FUNCTION_BLOCK "WEST_UHC126U_PFN"
TITLE =PN Driver
AUTHOR : 'W.E.St.'
VERSION : 1.1


VAR_INPUT
  DIRECT : BOOL ;	//Direktmodus (Sollwerte) / Direct mode for command position
  FF_ENABLE : BOOL ;	//Aktivierung der Vorsteuerung / Activation of the speed intrusion
  A_ENABLE : BOOL ;	//Aktivierung Beschleunigungsrückführung / Activation of the active damping press
  HAND_B : BOOL ;	//Handbefehl B / Manual command B
  HAND_A : BOOL ;	//Handbefehl A / Manual command A
  START : BOOL ;	//Startsignal Positionieren / Start positioning
  ENABLE : BOOL ;	//Freigabe / Unblocking
  PQ_ONLY : BOOL ;	//Deaktivierung Positionsregelung / deactivate position control
  PQ_SEL : BOOL ;	//Umschaltung zwischen Parametersatz 1 (false) und 2 (true) / Switching between p
  PQ_INVERSE : BOOL ;	//Umkehrung der Wirkrichtung des Druckreglers / Inverse mode of the pressure limi
  PQ_ACTIVE : BOOL ;	//Aktivieren des Druckreglers / Activation of the pressure limitation control
  DC_F_POS : BOOL ;	//Feinpositionierung / Fine positioning
  DC_ACTIVE : BOOL ;	//Driftkompensation / Drift compensation
  DC_FREEZE : BOOL ;	//Driftkompensation halten / Hold drift compensation value
  WA1 : REAL ;	//Sollposition 1 [mm] / Command position 1
  VA1 : REAL  := 1.000000e+002;	//Sollgeschwindigkeit 1 [%] / Command speed 1
  WA2 : REAL ;	//Sollposition 2 [mm] / Command position 2
  VA2 : REAL ;	//Sollgeschwindigkeit 2 [%] / Command speed 2
  WAP : REAL ;	//Solldruck [bar] / Command pressure
  PAR_CHANGE_IN : STRUCT
   ADDRESS : WORD ;
   PARVAL : DWORD ;
   PARAMODE : BOOL ;
   PARAVALID : BOOL ;
  END_STRUCT ;
  ADR_IN : INT ;	//Eingangsadresse des Slaves / Input adress of the slave
  ADR_OUT : INT ;	//Ausgangsadresse des Slaves / Output adress of the slave
END_VAR
VAR_OUTPUT
  PROFIL_2 : BOOL ;	//zweite Geschwindigkeit (Position) aktiv / 2nd speed (position) segment is activ
  POSWIN_S : BOOL ;	//Zielpositionsfenster erreicht / System within the target window
  POSWIN_D : BOOL ;	//Achse im Schleppfehlerfenster / following error within the window
  READY : BOOL ;	//Allgemeine Betriebsbereitschaft / operational readiness
  PRESSWIN : BOOL ;	//Druckistwert innerhalb des Drucksollwertfensters / Pressure control error withi
  PQ_ACTIVE_FB : BOOL ;	//Druckregler ist aktiv, hat Regelung übernommen / Pressure limitation control is
  PERROR1 : BOOL ;	//Fehler Drucksensor 1 / Error pressure sensor 1
  PERROR2 : BOOL ;	//Fehler Drucksensor 2 / Error pressure sensor 2
  SSIERROR : BOOL ;	//Fehler Wegmesssystem (SSI) / Error position sensor (SSI)
  XERROR : BOOL ;	//Fehler Wegmesssystem (analog) / Error position sensor (analogue)
  BUS_ERROR_CODE : BYTE ;	//Fehlercode zur Diagnose / Error code for diagnosis
  BUS_VALID : BOOL ;	//Buskopplung liefert gültige Werte / Bus Connection delivers valid information
  X : REAL ;	//Istposition [mm] / actual position
  W : REAL ;	//Interner Sollwert [mm] / Internal command position
  E : REAL ;	//Regelabweichung Position [mm] / actual position axis 2
  XDP : REAL ;	//Pseudo - Differenzdruck[bar] / Pseudo differential pressure
  X1 : REAL ;	//Druck X1 [bar] / Pressure X1
  X2 : REAL ;	//Druck X2 [bar] / Pressure X2
  ADD_OUT1 : REAL ;	//zusätzliches Ausgangssignal 1 / additional output 1
  ADD_OUT2 : REAL ;	//zusätzliches Ausgangssignal 2 / additional output 2
  PAR_CHANGE_OUT : STRUCT
   PARA_READY : BOOL ;
   PARA_ACTIVE : BOOL ;
  END_STRUCT ;
END_VAR
VAR
  DATA_IN : ARRAY  [0 .. 31 ] OF BYTE ;
  DATA_OUT : ARRAY  [0 .. 31 ] OF BYTE ;
  LIVEBIT : BOOL ;
  ERROR_TIMER_ON : INT ;
  ERROR_TIMER_OFF : INT ;
  i : INT ;	//Schleifenzähler
END_VAR
VAR_TEMP
  RET_VAL_TMP : INT ;
  TMP_VAL : DWORD ;
  TMP_VAL_WORD : WORD ;
  TMP_BYTE : BYTE ;
  TMP_VAL_REAL : REAL ;
  RCV_ERROR : BOOL ;
  SND_ERROR : BOOL ;
  LIVEBIT_ERROR : BOOL ;
  BUFFERR0V : BOOL ;
  CHKERROR : BOOL ;
  DERROR : BOOL ;
  LIVEBIT_FB : BOOL ;
  ADRE : WORD ;
END_VAR
BEGIN
NETWORK

      SET   ;
      SAVE  ;
      =     L     18.1;
      L     #ADR_IN;
      T     #ADRE;
      SAVE  ;
           CALL SFC   14 (
           LADDR                    := #ADRE,
           RET_VAL                  := #RET_VAL_TMP,
           RECORD                   := #DATA_IN);
      L     #RET_VAL_TMP;
      L     0;
      <>I   ;
      =     #RCV_ERROR;
      L     #DATA_IN[0];
      T     #TMP_BYTE;
      U     L      8.4;
      =     #PROFIL_2;
      U     L      8.5;
      =     #POSWIN_S;
      U     L      8.6;
      =     #POSWIN_D;
      U     L      8.7;
      =     #READY;
      L     #DATA_IN[1];
      T     #TMP_BYTE;
      U     L      8.6;
      =     #PRESSWIN;
      U     L      8.7;
      =     #PQ_ACTIVE_FB;
      L     #DATA_IN[2];
      T     #TMP_BYTE;
      U     L      8.1;
      NOT   ;
      =     #PERROR2;
      U     L      8.2;
      NOT   ;
      =     #PERROR1;
      U     L      8.3;
      NOT   ;
      =     #SSIERROR;
      U     L      8.4;
      NOT   ;
      =     #XERROR;
      U     L      8.5;
      NOT   ;
      =     #BUFFERR0V;
      U     L      8.6;
      NOT   ;
      =     #CHKERROR;
      U     L      8.7;
      NOT   ;
      =     #DERROR;
      L     #DATA_IN[3];
      T     #TMP_BYTE;
      U     L      8.0;
      =     #LIVEBIT_FB;
      U     L      8.6;
      =     #PAR_CHANGE_OUT.PARA_READY;
      U     L      8.7;
      =     #PAR_CHANGE_OUT.PARA_ACTIVE;
      U     #LIVEBIT;
      X     #LIVEBIT_FB;
      SPBN  A7d0;
      L     #ERROR_TIMER_ON;
      L     1;
      +I    ;
      SPO   I007;
      SPA   I008;
I007: CLR   ;
      =     L     18.1;
I008: T     #ERROR_TIMER_ON;
      SPA   A7d1;
A7d0: CLR   ;
      U     #LIVEBIT;
      NOT   ;
      =     #LIVEBIT;
      L     0;
      T     #ERROR_TIMER_ON;
A7d1: L     #ERROR_TIMER_ON;
      L     10;
      >=I   ;
      SPBN  A7d2;
      U     #LIVEBIT;
      NOT   ;
      =     #LIVEBIT;
      L     0;
      T     #ERROR_TIMER_ON;
      L     25;
      T     #ERROR_TIMER_OFF;
A7d2: L     #ERROR_TIMER_OFF;
      L     0;
      >I    ;
      SPBN  A7d3;
      L     #ERROR_TIMER_OFF;
      L     1;
      -I    ;
      SPO   I009;
      SPA   I00a;
I009: CLR   ;
      =     L     18.1;
I00a: T     #ERROR_TIMER_OFF;
      SET   ;
      =     #LIVEBIT_ERROR;
      SPA   A7d4;
A7d3: CLR   ;
      =     #LIVEBIT_ERROR;
A7d4: L     0;
      T     #i;
A7d5: L     #i;
      L     3;
      <=I   ;
      SPBN  A7d6;
      L     1;
      L     #i;
      +I    ;
      SPO   I00b;
      SPA   I00c;
I00b: CLR   ;
      =     L     18.1;
I00c: ITD   ;
      L     L#1;
      >=D   ;
      U     L     18.1;
      =     L     18.1;
      TAK   ;
      L     L#4;
      <=D   ;
      U     L     18.1;
      =     L     18.1;
      TAK   ;
      L     L#1;
      -D    ;
      SPO   I00d;
      SPA   I00e;
I00d: CLR   ;
      =     L     18.1;
I00e: L     L#8;
      *D    ;
      SPO   I00f;
      SPA   I010;
I00f: CLR   ;
      =     L     18.1;
I010: L     4;
      TAK   ;
      T     LD    20;
      TAK   ;
      L     #i;
      +I    ;
      SPO   I011;
      SPA   I012;
I011: CLR   ;
      =     L     18.1;
I012: ITD   ;
      L     L#0;
      >=D   ;
      U     L     18.1;
      =     L     18.1;
      TAK   ;
      L     L#31;
      <=D   ;
      U     L     18.1;
      =     L     18.1;
      TAK   ;
      L     L#8;
      *D    ;
      SPO   I013;
      SPA   I014;
I013: CLR   ;
      =     L     18.1;
I014: TAR2  ;
      +D    ;
      SPO   I015;
      SPA   I016;
I015: CLR   ;
      =     L     18.1;
I016: LAR1  ;
      L     DIB [AR1,P#72.0];
      LAR1  LD    20;
      T     LB [AR1,P#2.0];
      L     #i;
      L     1;
      +I    ;
      SPO   I017;
      SPA   I018;
I017: CLR   ;
      =     L     18.1;
I018: T     #i;
      SPA   A7d5;
A7d6: L     #TMP_VAL;
      CLR   ;
      U     L     18.1;
      SAVE  ;
      DTR   ;
      SAVE  ;
      L     1.000000e+003;
      /R    ;
      SPO   I019;
      SPA   I01a;
I019: CLR   ;
      =     L     18.1;
I01a: T     #X;
      L     0;
      T     #i;
A7d7: L     #i;
      L     3;
      <=I   ;
      SPBN  A7d8;
      L     1;
      L     #i;
      +I    ;
      SPO   I01b;
      SPA   I01c;
I01b: CLR   ;
      =     L     18.1;
I01c: ITD   ;
      L     L#1;
      >=D   ;
      U     L     18.1;
      =     L     18.1;
      TAK   ;
      L     L#4;
      <=D   ;
      U     L     18.1;
      =     L     18.1;
      TAK   ;
      L     L#1;
      -D    ;
      SPO   I01d;
      SPA   I01e;
I01d: CLR   ;
      =     L     18.1;
I01e: L     L#8;
      *D    ;
      SPO   I01f;
      SPA   I020;
I01f: CLR   ;
      =     L     18.1;
I020: L     8;
      TAK   ;
      T     LD    20;
      TAK   ;
      L     #i;
      +I    ;
      SPO   I021;
      SPA   I022;
I021: CLR   ;
      =     L     18.1;
I022: ITD   ;
      L     L#0;
      >=D   ;
      U     L     18.1;
      =     L     18.1;
      TAK   ;
      L     L#31;
      <=D   ;
      U     L     18.1;
      =     L     18.1;
      TAK   ;
      L     L#8;
      *D    ;
      SPO   I023;
      SPA   I024;
I023: CLR   ;
      =     L     18.1;
I024: TAR2  ;
      +D    ;
      SPO   I025;
      SPA   I026;
I025: CLR   ;
      =     L     18.1;
I026: LAR1  ;
      L     DIB [AR1,P#72.0];
      LAR1  LD    20;
      T     LB [AR1,P#2.0];
      L     #i;
      L     1;
      +I    ;
      SPO   I027;
      SPA   I028;
I027: CLR   ;
      =     L     18.1;
I028: T     #i;
      SPA   A7d7;
A7d8: L     #TMP_VAL;
      CLR   ;
      U     L     18.1;
      SAVE  ;
      DTR   ;
      SAVE  ;
      L     1.000000e+003;
      /R    ;
      SPO   I029;
      SPA   I02a;
I029: CLR   ;
      =     L     18.1;
I02a: T     #W;
      L     0;
      T     #i;
A7d9: L     #i;
      L     3;
      <=I   ;
      SPBN  A7da;
      L     1;
      L     #i;
      +I    ;
      SPO   I02b;
      SPA   I02c;
I02b: CLR   ;
      =     L     18.1;
I02c: ITD   ;
      L     L#1;
      >=D   ;
      U     L     18.1;
      =     L     18.1;
      TAK   ;
      L     L#4;
      <=D   ;
      U     L     18.1;
      =     L     18.1;
      TAK   ;
      L     L#1;
      -D    ;
      SPO   I02d;
      SPA   I02e;
I02d: CLR   ;
      =     L     18.1;
I02e: L     L#8;
      *D    ;
      SPO   I02f;
      SPA   I030;
I02f: CLR   ;
      =     L     18.1;
I030: L     12;
      TAK   ;
      T     LD    20;
      TAK   ;
      L     #i;
      +I    ;
      SPO   I031;
      SPA   I032;
I031: CLR   ;
      =     L     18.1;
I032: ITD   ;
      L     L#0;
      >=D   ;
      U     L     18.1;
      =     L     18.1;
      TAK   ;
      L     L#31;
      <=D   ;
      U     L     18.1;
      =     L     18.1;
      TAK   ;
      L     L#8;
      *D    ;
      SPO   I033;
      SPA   I034;
I033: CLR   ;
      =     L     18.1;
I034: TAR2  ;
      +D    ;
      SPO   I035;
      SPA   I036;
I035: CLR   ;
      =     L     18.1;
I036: LAR1  ;
      L     DIB [AR1,P#72.0];
      LAR1  LD    20;
      T     LB [AR1,P#2.0];
      L     #i;
      L     1;
      +I    ;
      SPO   I037;
      SPA   I038;
I037: CLR   ;
      =     L     18.1;
I038: T     #i;
      SPA   A7d9;
A7da: L     #TMP_VAL;
      CLR   ;
      U     L     18.1;
      SAVE  ;
      DTR   ;
      SAVE  ;
      L     1.000000e+003;
      /R    ;
      SPO   I039;
      SPA   I03a;
I039: CLR   ;
      =     L     18.1;
I03a: T     #E;
      L     0;
      T     #i;
A7db: L     #i;
      L     1;
      <=I   ;
      SPBN  A7dc;
      L     #i;
      +I    ;
      SPO   I03b;
      SPA   I03c;
I03b: CLR   ;
      =     L     18.1;
I03c: ITD   ;
      L     L#1;
      >=D   ;
      U     L     18.1;
      =     L     18.1;
      TAK   ;
      L     L#2;
      <=D   ;
      U     L     18.1;
      =     L     18.1;
      TAK   ;
      L     L#1;
      -D    ;
      SPO   I03d;
      SPA   I03e;
I03d: CLR   ;
      =     L     18.1;
I03e: L     L#8;
      *D    ;
      SPO   I03f;
      SPA   I040;
I03f: CLR   ;
      =     L     18.1;
I040: L     16;
      TAK   ;
      T     LD    20;
      TAK   ;
      L     #i;
      +I    ;
      SPO   I041;
      SPA   I042;
I041: CLR   ;
      =     L     18.1;
I042: ITD   ;
      L     L#0;
      >=D   ;
      U     L     18.1;
      =     L     18.1;
      TAK   ;
      L     L#31;
      <=D   ;
      U     L     18.1;
      =     L     18.1;
      TAK   ;
      L     L#8;
      *D    ;
      SPO   I043;
      SPA   I044;
I043: CLR   ;
      =     L     18.1;
I044: TAR2  ;
      +D    ;
      SPO   I045;
      SPA   I046;
I045: CLR   ;
      =     L     18.1;
I046: LAR1  ;
      L     DIB [AR1,P#72.0];
      LAR1  LD    20;
      T     LB [AR1,P#6.0];
      L     #i;
      L     1;
      +I    ;
      SPO   I047;
      SPA   I048;
I047: CLR   ;
      =     L     18.1;
I048: T     #i;
      SPA   A7db;
A7dc: L     #TMP_VAL_WORD;
      CLR   ;
      U     L     18.1;
      SAVE  ;
      ITD   ;
      DTR   ;
      T     #TMP_VAL_REAL;
      SAVE  ;
      L     1.000000e+001;
      /R    ;
      SPO   I049;
      SPA   I04a;
I049: CLR   ;
      =     L     18.1;
I04a: T     #XDP;
      L     0;
      T     #i;
A7dd: L     #i;
      L     1;
      <=I   ;
      SPBN  A7de;
      L     #i;
      +I    ;
      SPO   I04b;
      SPA   I04c;
I04b: CLR   ;
      =     L     18.1;
I04c: ITD   ;
      L     L#1;
      >=D   ;
      U     L     18.1;
      =     L     18.1;
      TAK   ;
      L     L#2;
      <=D   ;
      U     L     18.1;
      =     L     18.1;
      TAK   ;
      L     L#1;
      -D    ;
      SPO   I04d;
      SPA   I04e;
I04d: CLR   ;
      =     L     18.1;
I04e: L     L#8;
      *D    ;
      SPO   I04f;
      SPA   I050;
I04f: CLR   ;
      =     L     18.1;
I050: L     18;
      TAK   ;
      T     LD    20;
      TAK   ;
      L     #i;
      +I    ;
      SPO   I051;
      SPA   I052;
I051: CLR   ;
      =     L     18.1;
I052: ITD   ;
      L     L#0;
      >=D   ;
      U     L     18.1;
      =     L     18.1;
      TAK   ;
      L     L#31;
      <=D   ;
      U     L     18.1;
      =     L     18.1;
      TAK   ;
      L     L#8;
      *D    ;
      SPO   I053;
      SPA   I054;
I053: CLR   ;
      =     L     18.1;
I054: TAR2  ;
      +D    ;
      SPO   I055;
      SPA   I056;
I055: CLR   ;
      =     L     18.1;
I056: LAR1  ;
      L     DIB [AR1,P#72.0];
      LAR1  LD    20;
      T     LB [AR1,P#6.0];
      L     #i;
      L     1;
      +I    ;
      SPO   I057;
      SPA   I058;
I057: CLR   ;
      =     L     18.1;
I058: T     #i;
      SPA   A7dd;
A7de: L     #TMP_VAL_WORD;
      CLR   ;
      U     L     18.1;
      SAVE  ;
      ITD   ;
      DTR   ;
      T     #TMP_VAL_REAL;
      SAVE  ;
      L     1.000000e+001;
      /R    ;
      SPO   I059;
      SPA   I05a;
I059: CLR   ;
      =     L     18.1;
I05a: T     #X1;
      L     0;
      T     #i;
A7df: L     #i;
      L     1;
      <=I   ;
      SPBN  A7e0;
      L     #i;
      +I    ;
      SPO   I05b;
      SPA   I05c;
I05b: CLR   ;
      =     L     18.1;
I05c: ITD   ;
      L     L#1;
      >=D   ;
      U     L     18.1;
      =     L     18.1;
      TAK   ;
      L     L#2;
      <=D   ;
      U     L     18.1;
      =     L     18.1;
      TAK   ;
      L     L#1;
      -D    ;
      SPO   I05d;
      SPA   I05e;
I05d: CLR   ;
      =     L     18.1;
I05e: L     L#8;
      *D    ;
      SPO   I05f;
      SPA   I060;
I05f: CLR   ;
      =     L     18.1;
I060: L     20;
      TAK   ;
      T     LD    20;
      TAK   ;
      L     #i;
      +I    ;
      SPO   I061;
      SPA   I062;
I061: CLR   ;
      =     L     18.1;
I062: ITD   ;
      L     L#0;
      >=D   ;
      U     L     18.1;
      =     L     18.1;
      TAK   ;
      L     L#31;
      <=D   ;
      U     L     18.1;
      =     L     18.1;
      TAK   ;
      L     L#8;
      *D    ;
      SPO   I063;
      SPA   I064;
I063: CLR   ;
      =     L     18.1;
I064: TAR2  ;
      +D    ;
      SPO   I065;
      SPA   I066;
I065: CLR   ;
      =     L     18.1;
I066: LAR1  ;
      L     DIB [AR1,P#72.0];
      LAR1  LD    20;
      T     LB [AR1,P#6.0];
      L     #i;
      L     1;
      +I    ;
      SPO   I067;
      SPA   I068;
I067: CLR   ;
      =     L     18.1;
I068: T     #i;
      SPA   A7df;
A7e0: L     #TMP_VAL_WORD;
      CLR   ;
      U     L     18.1;
      SAVE  ;
      ITD   ;
      DTR   ;
      T     #TMP_VAL_REAL;
      SAVE  ;
      L     1.000000e+001;
      /R    ;
      SPO   I069;
      SPA   I06a;
I069: CLR   ;
      =     L     18.1;
I06a: T     #X2;
      L     0;
      T     #i;
A7e1: L     #i;
      L     1;
      <=I   ;
      SPBN  A7e2;
      L     #i;
      +I    ;
      SPO   I06b;
      SPA   I06c;
I06b: CLR   ;
      =     L     18.1;
I06c: ITD   ;
      L     L#1;
      >=D   ;
      U     L     18.1;
      =     L     18.1;
      TAK   ;
      L     L#2;
      <=D   ;
      U     L     18.1;
      =     L     18.1;
      TAK   ;
      L     L#1;
      -D    ;
      SPO   I06d;
      SPA   I06e;
I06d: CLR   ;
      =     L     18.1;
I06e: L     L#8;
      *D    ;
      SPO   I06f;
      SPA   I070;
I06f: CLR   ;
      =     L     18.1;
I070: L     22;
      TAK   ;
      T     LD    20;
      TAK   ;
      L     #i;
      +I    ;
      SPO   I071;
      SPA   I072;
I071: CLR   ;
      =     L     18.1;
I072: ITD   ;
      L     L#0;
      >=D   ;
      U     L     18.1;
      =     L     18.1;
      TAK   ;
      L     L#31;
      <=D   ;
      U     L     18.1;
      =     L     18.1;
      TAK   ;
      L     L#8;
      *D    ;
      SPO   I073;
      SPA   I074;
I073: CLR   ;
      =     L     18.1;
I074: TAR2  ;
      +D    ;
      SPO   I075;
      SPA   I076;
I075: CLR   ;
      =     L     18.1;
I076: LAR1  ;
      L     DIB [AR1,P#72.0];
      LAR1  LD    20;
      T     LB [AR1,P#6.0];
      L     #i;
      L     1;
      +I    ;
      SPO   I077;
      SPA   I078;
I077: CLR   ;
      =     L     18.1;
I078: T     #i;
      SPA   A7e1;
A7e2: L     #TMP_VAL_WORD;
      CLR   ;
      U     L     18.1;
      SAVE  ;
      ITD   ;
      DTR   ;
      T     #ADD_OUT1;
      SAVE  ;
      L     0;
      T     #i;
A7e3: L     #i;
      L     1;
      <=I   ;
      SPBN  A7e4;
      L     #i;
      +I    ;
      SPO   I079;
      SPA   I07a;
I079: CLR   ;
      =     L     18.1;
I07a: ITD   ;
      L     L#1;
      >=D   ;
      U     L     18.1;
      =     L     18.1;
      TAK   ;
      L     L#2;
      <=D   ;
      U     L     18.1;
      =     L     18.1;
      TAK   ;
      L     L#1;
      -D    ;
      SPO   I07b;
      SPA   I07c;
I07b: CLR   ;
      =     L     18.1;
I07c: L     L#8;
      *D    ;
      SPO   I07d;
      SPA   I07e;
I07d: CLR   ;
      =     L     18.1;
I07e: L     24;
      TAK   ;
      T     LD    20;
      TAK   ;
      L     #i;
      +I    ;
      SPO   I07f;
      SPA   I080;
I07f: CLR   ;
      =     L     18.1;
I080: ITD   ;
      L     L#0;
      >=D   ;
      U     L     18.1;
      =     L     18.1;
      TAK   ;
      L     L#31;
      <=D   ;
      U     L     18.1;
      =     L     18.1;
      TAK   ;
      L     L#8;
      *D    ;
      SPO   I081;
      SPA   I082;
I081: CLR   ;
      =     L     18.1;
I082: TAR2  ;
      +D    ;
      SPO   I083;
      SPA   I084;
I083: CLR   ;
      =     L     18.1;
I084: LAR1  ;
      L     DIB [AR1,P#72.0];
      LAR1  LD    20;
      T     LB [AR1,P#6.0];
      L     #i;
      L     1;
      +I    ;
      SPO   I085;
      SPA   I086;
I085: CLR   ;
      =     L     18.1;
I086: T     #i;
      SPA   A7e3;
A7e4: L     #TMP_VAL_WORD;
      CLR   ;
      U     L     18.1;
      SAVE  ;
      ITD   ;
      DTR   ;
      T     #ADD_OUT2;
      SAVE  ;
      CLR   ;
      U     #DIRECT;
      =     L      8.0;
      U     #FF_ENABLE;
      =     L      8.1;
      U     #A_ENABLE;
      =     L      8.2;
      CLR   ;
      =     L      8.3;
      U     #HAND_B;
      =     L      8.4;
      U     #HAND_A;
      =     L      8.5;
      U     #START;
      =     L      8.6;
      U     #ENABLE;
      =     L      8.7;
      L     #TMP_BYTE;
      T     #DATA_OUT[0];
      CLR   ;
      =     L      8.0;
      =     L      8.1;
      =     L      8.2;
      =     L      8.3;
      U     #PQ_ONLY;
      =     L      8.4;
      U     #PQ_SEL;
      =     L      8.5;
      U     #PQ_INVERSE;
      =     L      8.6;
      U     #PQ_ACTIVE;
      =     L      8.7;
      L     #TMP_BYTE;
      T     #DATA_OUT[1];
      U     #LIVEBIT;
      =     L      8.0;
      CLR   ;
      =     L      8.1;
      =     L      8.2;
      =     L      8.3;
      =     L      8.4;
      U     #DC_FREEZE;
      =     L      8.5;
      U     #DC_ACTIVE;
      =     L      8.6;
      U     #DC_F_POS;
      =     L      8.7;
      L     #TMP_BYTE;
      T     #DATA_OUT[2];
      CLR   ;
      =     L      8.0;
      =     L      8.1;
      =     L      8.2;
      =     L      8.3;
      =     L      8.4;
      =     L      8.5;
      U     #PAR_CHANGE_IN.PARAVALID;
      =     L      8.6;
      U     #PAR_CHANGE_IN.PARAMODE;
      =     L      8.7;
      L     #TMP_BYTE;
      T     #DATA_OUT[3];
      L     #WA1;
      L     1.000000e+003;
      *R    ;
      SPO   I087;
      SPA   I088;
I087: CLR   ;
      =     L     18.1;
I088: RND   ;
      SPO   I089;
      SPA   I08a;
I089: CLR   ;
      =     L     18.1;
I08a: CLR   ;
      U     L     18.1;
      SAVE  ;
      T     #TMP_VAL;
      SAVE  ;
      L     0;
      T     #i;
A7e5: L     #i;
      L     3;
      <=I   ;
      SPBN  A7e6;
      L     4;
      L     #i;
      +I    ;
      SPO   I08b;
      SPA   I08c;
I08b: CLR   ;
      =     L     18.1;
I08c: ITD   ;
      L     L#0;
      >=D   ;
      U     L     18.1;
      =     L     18.1;
      TAK   ;
      L     L#31;
      <=D   ;
      U     L     18.1;
      =     L     18.1;
      TAK   ;
      L     L#8;
      *D    ;
      SPO   I08d;
      SPA   I08e;
I08d: CLR   ;
      =     L     18.1;
I08e: TAR2  ;
      +D    ;
      SPO   I08f;
      SPA   I090;
I08f: CLR   ;
      =     L     18.1;
I090: L     1;
      TAK   ;
      T     LD    20;
      TAK   ;
      L     #i;
      +I    ;
      SPO   I091;
      SPA   I092;
I091: CLR   ;
      =     L     18.1;
I092: ITD   ;
      L     L#1;
      >=D   ;
      U     L     18.1;
      =     L     18.1;
      TAK   ;
      L     L#4;
      <=D   ;
      U     L     18.1;
      =     L     18.1;
      TAK   ;
      L     L#1;
      -D    ;
      SPO   I093;
      SPA   I094;
I093: CLR   ;
      =     L     18.1;
I094: L     L#8;
      *D    ;
      SPO   I095;
      SPA   I096;
I095: CLR   ;
      =     L     18.1;
I096: LAR1  ;
      L     LB [AR1,P#2.0];
      LAR1  LD    20;
      T     DIB [AR1,P#104.0];
      L     #i;
      L     1;
      +I    ;
      SPO   I097;
      SPA   I098;
I097: CLR   ;
      =     L     18.1;
I098: T     #i;
      SPA   A7e5;
A7e6: L     #VA1;
      T     #TMP_VAL_REAL;
      L     0.000000e+000;
      <R    ;
      =     L     18.2;
      U     #PQ_ACTIVE;
      NOT   ;
      U     L     18.2;
      SPBN  A7e7;
      T     #TMP_VAL_REAL;
      SPA   A7e9;
A7e7: L     #TMP_VAL_REAL;
      L     -1.000000e+002;
      <R    ;
      SPBN  A7e9;
      T     #TMP_VAL_REAL;
A7e9: L     #TMP_VAL_REAL;
      L     1.000000e+002;
      >R    ;
      SPBN  A7ea;
      T     #TMP_VAL_REAL;
A7ea: L     #TMP_VAL_REAL;
      L     1.638300e+002;
      *R    ;
      SPO   I099;
      SPA   I09a;
I099: CLR   ;
      =     L     18.1;
I09a: T     #TMP_VAL_REAL;
      RND   ;
      SPO   I09b;
      SPA   I09c;
I09b: CLR   ;
      =     L     18.1;
I09c: CLR   ;
      U     L     18.1;
      SAVE  ;
      T     #TMP_VAL;
      SAVE  ;
      L     0;
      T     #i;
A7eb: L     #i;
      L     1;
      <=I   ;
      SPBN  A7ec;
      L     8;
      L     #i;
      +I    ;
      SPO   I09d;
      SPA   I09e;
I09d: CLR   ;
      =     L     18.1;
I09e: ITD   ;
      L     L#0;
      >=D   ;
      U     L     18.1;
      =     L     18.1;
      TAK   ;
      L     L#31;
      <=D   ;
      U     L     18.1;
      =     L     18.1;
      TAK   ;
      L     L#8;
      *D    ;
      SPO   I09f;
      SPA   I0a0;
I09f: CLR   ;
      =     L     18.1;
I0a0: TAR2  ;
      +D    ;
      SPO   I0a1;
      SPA   I0a2;
I0a1: CLR   ;
      =     L     18.1;
I0a2: L     3;
      TAK   ;
      T     LD    20;
      TAK   ;
      L     #i;
      +I    ;
      SPO   I0a3;
      SPA   I0a4;
I0a3: CLR   ;
      =     L     18.1;
I0a4: ITD   ;
      L     L#1;
      >=D   ;
      U     L     18.1;
      =     L     18.1;
      TAK   ;
      L     L#4;
      <=D   ;
      U     L     18.1;
      =     L     18.1;
      TAK   ;
      L     L#1;
      -D    ;
      SPO   I0a5;
      SPA   I0a6;
I0a5: CLR   ;
      =     L     18.1;
I0a6: L     L#8;
      *D    ;
      SPO   I0a7;
      SPA   I0a8;
I0a7: CLR   ;
      =     L     18.1;
I0a8: LAR1  ;
      L     LB [AR1,P#2.0];
      LAR1  LD    20;
      T     DIB [AR1,P#104.0];
      L     #i;
      L     1;
      +I    ;
      SPO   I0a9;
      SPA   I0aa;
I0a9: CLR   ;
      =     L     18.1;
I0aa: T     #i;
      SPA   A7eb;
A7ec: L     #WA2;
      L     1.000000e+003;
      *R    ;
      SPO   I0ab;
      SPA   I0ac;
I0ab: CLR   ;
      =     L     18.1;
I0ac: RND   ;
      SPO   I0ad;
      SPA   I0ae;
I0ad: CLR   ;
      =     L     18.1;
I0ae: CLR   ;
      U     L     18.1;
      SAVE  ;
      T     #TMP_VAL;
      SAVE  ;
      L     0;
      T     #i;
A7ed: L     #i;
      L     3;
      <=I   ;
      SPBN  A7ee;
      L     10;
      L     #i;
      +I    ;
      SPO   I0af;
      SPA   I0b0;
I0af: CLR   ;
      =     L     18.1;
I0b0: ITD   ;
      L     L#0;
      >=D   ;
      U     L     18.1;
      =     L     18.1;
      TAK   ;
      L     L#31;
      <=D   ;
      U     L     18.1;
      =     L     18.1;
      TAK   ;
      L     L#8;
      *D    ;
      SPO   I0b1;
      SPA   I0b2;
I0b1: CLR   ;
      =     L     18.1;
I0b2: TAR2  ;
      +D    ;
      SPO   I0b3;
      SPA   I0b4;
I0b3: CLR   ;
      =     L     18.1;
I0b4: L     1;
      TAK   ;
      T     LD    20;
      TAK   ;
      L     #i;
      +I    ;
      SPO   I0b5;
      SPA   I0b6;
I0b5: CLR   ;
      =     L     18.1;
I0b6: ITD   ;
      L     L#1;
      >=D   ;
      U     L     18.1;
      =     L     18.1;
      TAK   ;
      L     L#4;
      <=D   ;
      U     L     18.1;
      =     L     18.1;
      TAK   ;
      L     L#1;
      -D    ;
      SPO   I0b7;
      SPA   I0b8;
I0b7: CLR   ;
      =     L     18.1;
I0b8: L     L#8;
      *D    ;
      SPO   I0b9;
      SPA   I0ba;
I0b9: CLR   ;
      =     L     18.1;
I0ba: LAR1  ;
      L     LB [AR1,P#2.0];
      LAR1  LD    20;
      T     DIB [AR1,P#104.0];
      L     #i;
      L     1;
      +I    ;
      SPO   I0bb;
      SPA   I0bc;
I0bb: CLR   ;
      =     L     18.1;
I0bc: T     #i;
      SPA   A7ed;
A7ee: L     #VA2;
      T     #TMP_VAL_REAL;
      L     0.000000e+000;
      <R    ;
      SPBN  A7ef;
      T     #TMP_VAL_REAL;
      SPA   A7f1;
A7ef: L     #TMP_VAL_REAL;
      L     1.000000e+002;
      >R    ;
      SPBN  A7f1;
      T     #TMP_VAL_REAL;
A7f1: L     #TMP_VAL_REAL;
      L     1.638300e+002;
      *R    ;
      SPO   I0bd;
      SPA   I0be;
I0bd: CLR   ;
      =     L     18.1;
I0be: T     #TMP_VAL_REAL;
      RND   ;
      SPO   I0bf;
      SPA   I0c0;
I0bf: CLR   ;
      =     L     18.1;
I0c0: CLR   ;
      U     L     18.1;
      SAVE  ;
      T     #TMP_VAL;
      SAVE  ;
      L     0;
      T     #i;
A7f2: L     #i;
      L     1;
      <=I   ;
      SPBN  A7f3;
      L     14;
      L     #i;
      +I    ;
      SPO   I0c1;
      SPA   I0c2;
I0c1: CLR   ;
      =     L     18.1;
I0c2: ITD   ;
      L     L#0;
      >=D   ;
      U     L     18.1;
      =     L     18.1;
      TAK   ;
      L     L#31;
      <=D   ;
      U     L     18.1;
      =     L     18.1;
      TAK   ;
      L     L#8;
      *D    ;
      SPO   I0c3;
      SPA   I0c4;
I0c3: CLR   ;
      =     L     18.1;
I0c4: TAR2  ;
      +D    ;
      SPO   I0c5;
      SPA   I0c6;
I0c5: CLR   ;
      =     L     18.1;
I0c6: L     3;
      TAK   ;
      T     LD    20;
      TAK   ;
      L     #i;
      +I    ;
      SPO   I0c7;
      SPA   I0c8;
I0c7: CLR   ;
      =     L     18.1;
I0c8: ITD   ;
      L     L#1;
      >=D   ;
      U     L     18.1;
      =     L     18.1;
      TAK   ;
      L     L#4;
      <=D   ;
      U     L     18.1;
      =     L     18.1;
      TAK   ;
      L     L#1;
      -D    ;
      SPO   I0c9;
      SPA   I0ca;
I0c9: CLR   ;
      =     L     18.1;
I0ca: L     L#8;
      *D    ;
      SPO   I0cb;
      SPA   I0cc;
I0cb: CLR   ;
      =     L     18.1;
I0cc: LAR1  ;
      L     LB [AR1,P#2.0];
      LAR1  LD    20;
      T     DIB [AR1,P#104.0];
      L     #i;
      L     1;
      +I    ;
      SPO   I0cd;
      SPA   I0ce;
I0cd: CLR   ;
      =     L     18.1;
I0ce: T     #i;
      SPA   A7f2;
A7f3: L     #WAP;
      T     #TMP_VAL_REAL;
      L     0.000000e+000;
      <R    ;
      SPBN  A7f4;
      T     #TMP_VAL_REAL;
      SPA   A7f6;
A7f4: L     #TMP_VAL_REAL;
      L     1.000000e+003;
      >R    ;
      SPBN  A7f6;
      T     #TMP_VAL_REAL;
A7f6: L     #TMP_VAL_REAL;
      L     1.000000e+001;
      *R    ;
      SPO   I0cf;
      SPA   I0d0;
I0cf: CLR   ;
      =     L     18.1;
I0d0: T     #TMP_VAL_REAL;
      RND   ;
      SPO   I0d1;
      SPA   I0d2;
I0d1: CLR   ;
      =     L     18.1;
I0d2: CLR   ;
      U     L     18.1;
      SAVE  ;
      T     #TMP_VAL;
      SAVE  ;
      L     0;
      T     #i;
A7f7: L     #i;
      L     1;
      <=I   ;
      SPBN  A7f8;
      L     16;
      L     #i;
      +I    ;
      SPO   I0d3;
      SPA   I0d4;
I0d3: CLR   ;
      =     L     18.1;
I0d4: ITD   ;
      L     L#0;
      >=D   ;
      U     L     18.1;
      =     L     18.1;
      TAK   ;
      L     L#31;
      <=D   ;
      U     L     18.1;
      =     L     18.1;
      TAK   ;
      L     L#8;
      *D    ;
      SPO   I0d5;
      SPA   I0d6;
I0d5: CLR   ;
      =     L     18.1;
I0d6: TAR2  ;
      +D    ;
      SPO   I0d7;
      SPA   I0d8;
I0d7: CLR   ;
      =     L     18.1;
I0d8: L     3;
      TAK   ;
      T     LD    20;
      TAK   ;
      L     #i;
      +I    ;
      SPO   I0d9;
      SPA   I0da;
I0d9: CLR   ;
      =     L     18.1;
I0da: ITD   ;
      L     L#1;
      >=D   ;
      U     L     18.1;
      =     L     18.1;
      TAK   ;
      L     L#4;
      <=D   ;
      U     L     18.1;
      =     L     18.1;
      TAK   ;
      L     L#1;
      -D    ;
      SPO   I0db;
      SPA   I0dc;
I0db: CLR   ;
      =     L     18.1;
I0dc: L     L#8;
      *D    ;
      SPO   I0dd;
      SPA   I0de;
I0dd: CLR   ;
      =     L     18.1;
I0de: LAR1  ;
      L     LB [AR1,P#2.0];
      LAR1  LD    20;
      T     DIB [AR1,P#104.0];
      L     #i;
      L     1;
      +I    ;
      SPO   I0df;
      SPA   I0e0;
I0df: CLR   ;
      =     L     18.1;
I0e0: T     #i;
      SPA   A7f7;
A7f8: L     #PAR_CHANGE_IN.ADDRESS;
      UD    DW#16#FFFF;
      T     #TMP_VAL;
      CLR   ;
      U     L     18.1;
      SAVE  ;
      L     0;
      T     #i;
A7f9: L     #i;
      L     1;
      <=I   ;
      SPBN  A7fa;
      L     30;
      L     #i;
      +I    ;
      SPO   I0e1;
      SPA   I0e2;
I0e1: CLR   ;
      =     L     18.1;
I0e2: ITD   ;
      L     L#0;
      >=D   ;
      U     L     18.1;
      =     L     18.1;
      TAK   ;
      L     L#31;
      <=D   ;
      U     L     18.1;
      =     L     18.1;
      TAK   ;
      L     L#8;
      *D    ;
      SPO   I0e3;
      SPA   I0e4;
I0e3: CLR   ;
      =     L     18.1;
I0e4: TAR2  ;
      +D    ;
      SPO   I0e5;
      SPA   I0e6;
I0e5: CLR   ;
      =     L     18.1;
I0e6: L     3;
      TAK   ;
      T     LD    20;
      TAK   ;
      L     #i;
      +I    ;
      SPO   I0e7;
      SPA   I0e8;
I0e7: CLR   ;
      =     L     18.1;
I0e8: ITD   ;
      L     L#1;
      >=D   ;
      U     L     18.1;
      =     L     18.1;
      TAK   ;
      L     L#4;
      <=D   ;
      U     L     18.1;
      =     L     18.1;
      TAK   ;
      L     L#1;
      -D    ;
      SPO   I0e9;
      SPA   I0ea;
I0e9: CLR   ;
      =     L     18.1;
I0ea: L     L#8;
      *D    ;
      SPO   I0eb;
      SPA   I0ec;
I0eb: CLR   ;
      =     L     18.1;
I0ec: LAR1  ;
      L     LB [AR1,P#2.0];
      LAR1  LD    20;
      T     DIB [AR1,P#104.0];
      L     #i;
      L     1;
      +I    ;
      SPO   I0ed;
      SPA   I0ee;
I0ed: CLR   ;
      =     L     18.1;
I0ee: T     #i;
      SPA   A7f9;
A7fa: L     #PAR_CHANGE_IN.PARVAL;
      T     #TMP_VAL;
      L     0;
      T     #i;
A7fb: L     #i;
      L     3;
      <=I   ;
      SPBN  A7fc;
      L     26;
      L     #i;
      +I    ;
      SPO   I0ef;
      SPA   I0f0;
I0ef: CLR   ;
      =     L     18.1;
I0f0: ITD   ;
      L     L#0;
      >=D   ;
      U     L     18.1;
      =     L     18.1;
      TAK   ;
      L     L#31;
      <=D   ;
      U     L     18.1;
      =     L     18.1;
      TAK   ;
      L     L#8;
      *D    ;
      SPO   I0f1;
      SPA   I0f2;
I0f1: CLR   ;
      =     L     18.1;
I0f2: TAR2  ;
      +D    ;
      SPO   I0f3;
      SPA   I0f4;
I0f3: CLR   ;
      =     L     18.1;
I0f4: L     1;
      TAK   ;
      T     LD    20;
      TAK   ;
      L     #i;
      +I    ;
      SPO   I0f5;
      SPA   I0f6;
I0f5: CLR   ;
      =     L     18.1;
I0f6: ITD   ;
      L     L#1;
      >=D   ;
      U     L     18.1;
      =     L     18.1;
      TAK   ;
      L     L#4;
      <=D   ;
      U     L     18.1;
      =     L     18.1;
      TAK   ;
      L     L#1;
      -D    ;
      SPO   I0f7;
      SPA   I0f8;
I0f7: CLR   ;
      =     L     18.1;
I0f8: L     L#8;
      *D    ;
      SPO   I0f9;
      SPA   I0fa;
I0f9: CLR   ;
      =     L     18.1;
I0fa: LAR1  ;
      L     LB [AR1,P#2.0];
      LAR1  LD    20;
      T     DIB [AR1,P#104.0];
      L     #i;
      L     1;
      +I    ;
      SPO   I0fb;
      SPA   I0fc;
I0fb: CLR   ;
      =     L     18.1;
I0fc: T     #i;
      SPA   A7fb;
A7fc: L     #ADR_OUT;
      T     #ADRE;
      CLR   ;
      U     L     18.1;
      SAVE  ;
	  CALL SFC   15 (
      LADDR                    := #ADRE,
      RECORD                   := #DATA_OUT,
      RET_VAL                  := #RET_VAL_TMP);
      L     #RET_VAL_TMP;
      L     0;
      <>I   ;
      =     #SND_ERROR;
      U     #DERROR;
      =     L      8.0;
      U     #CHKERROR;
      =     L      8.1;
      U     #BUFFERR0V;
      =     L      8.2;
      U     #RCV_ERROR;
      =     L      8.3;
      U     #SND_ERROR;
      =     L      8.4;
      U     #LIVEBIT_ERROR;
      =     L      8.5;
      CLR   ;
      =     L      8.6;
      =     L      8.7;
      L     #TMP_BYTE;
      T     #BUS_ERROR_CODE;
      L     B#16#0;
      ==I   ;
      =     #BUS_VALID;
      U     L     18.1;
      SAVE  ;
      BE    ;

END_FUNCTION_BLOCK

